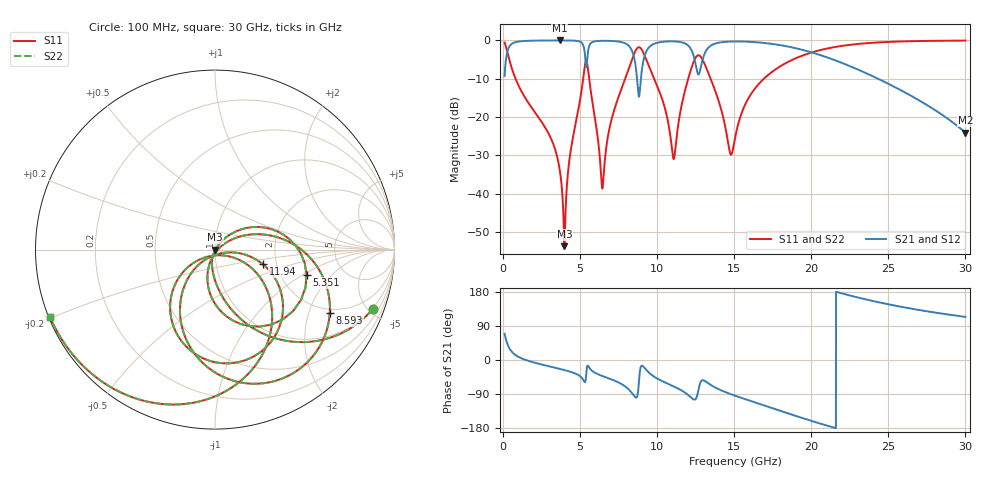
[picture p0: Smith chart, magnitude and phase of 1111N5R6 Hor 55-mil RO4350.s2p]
# GHz S MA R 50
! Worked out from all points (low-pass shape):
!   3201 points, 100 MHz to 30 GHz, reference 50 ohm
!   highest |S21| = -0.02 dB at 3.669 GHz (marker M1); lowest = -24.0 dB at 30 GHz (marker M2)
!   |S21| within 3 dB of the highest: 273.1 MHz to 5.294 GHz (5.021 GHz wide, 180 % of centre); 13.13 GHz to 19.93 GHz (6.797 GHz wide, 41.1 % of centre)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
!   lowest |S11| = -53.6 dB at 3.978 GHz (marker M3), VSWR 1.00, Z = 50.2 - j0.124 ohm
!   |S11| at or under -10 dB: 809.7 MHz to 5.201 GHz (4.391 GHz wide, 146 % of centre); 5.586 GHz to 7.922 GHz (2.337 GHz wide, 34.6 % of centre); 13.47 GHz to 16.92 GHz (3.454 GHz wide, 22.7 % of centre)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
!   |S22| runs from -53.6 to -0.1 dB; largest |S21 - S12| = 0
!   S11 on the Smith chart (normalised r, x): 100 MHz: 0.94, -5.30; 5.351 GHz: 2.78, -1.08; 8.593 GHz: 1.83, -2.77; 11.94 GHz: 1.70, -0.30; 30 GHz: 0.00, -0.20
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0.1  0.9392 -20.7  0.343 69.2  0.343 69.2  0.9392 -20.7
0.8568438  0.3 -78.2  0.9533 11.7  0.9533 11.7  0.3 -78.2
3.669313  0.02101 -109.1  0.9978 -23.3  0.9978 -23.3  0.02101 -109.1
3.977656  0.002079 -36.6  0.9975 -26.5  0.9975 -26.5  0.002079 -36.6
5.089563  0.2185 33.8  0.9379 -46.1  0.9379 -46.1  0.2185 33.8
5.351187  0.5293 -15.4  0.5336 -55.2  0.5336 -55.2  0.5293 -15.4
5.696906  0.214 -99.9  0.9199 -25.7  0.9199 -25.7  0.214 -99.9
6.45375  0.01185 -31.8  0.9876 -42.4  0.9876 -42.4  0.01185 -31.8
8.004812  0.3514 11.5  0.898 -72.3  0.898 -72.3  0.3514 11.5
8.593469  0.7306 -28.9  0.4741 -98.7  0.4741 -98.7  0.7306 -28.9
8.99525  0.7577 -78.3  0.3938 -15.1  0.3938 -15.1  0.7577 -78.3
10.06978  0.236 -132.2  0.9369 -50.5  0.9369 -50.5  0.236 -132.2
11.06956  0.0284 -73.2  0.9705 -69.7  0.9705 -69.7  0.0284 -73.2
11.93853  0.2793 -17.0  0.8813 -90.2  0.8813 -90.2  0.2793 -17.0
12.40572  0.5479 -48.0  0.5852 -104.5  0.5852 -104.5  0.5479 -48.0
12.82619  0.6121 -95.4  0.4426 -57.4  0.4426 -57.4  0.6121 -95.4
14.73231  0.03397 -102.5  0.9653 -89.4  0.9653 -89.4  0.03397 -102.5
15.05  0.05296 -37.5  0.9683 -94.1  0.9683 -94.1  0.05296 -37.5
16.58237  0.269 -29.6  0.9403 -115.1  0.9403 -115.1  0.269 -29.6
20.03956  0.6976 -72.6  0.6958 -161.1  0.6958 -161.1  0.6976 -72.6
25.01978  0.9552 -124.2  0.2706 146.8  0.2706 146.8  0.9552 -124.2
30  0.9934 -157.8  0.06275 113.7  0.06275 113.7  0.9934 -157.8
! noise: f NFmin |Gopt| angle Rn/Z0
0.1  0.001101  0.84  3.224  0.001457
3.417  0.009511  0.4687  23.48  0.002918
6.743  0.03593  0.6892  43.9  0.01945
10.06  0.07896  0.7839  64.4  0.05406
13.39  0.1745  0.8672  82.88  0.1595
16.7  0.07861  0.6768  98.8  0.02089
20.03  0.09342  0.6871  112.5  0.01929
23.35  0.1359  0.7615  126.7  0.02494
26.67  0.2403  0.8581  142.5  0.03929
30  0.6029  0.9425  159  0.07995
